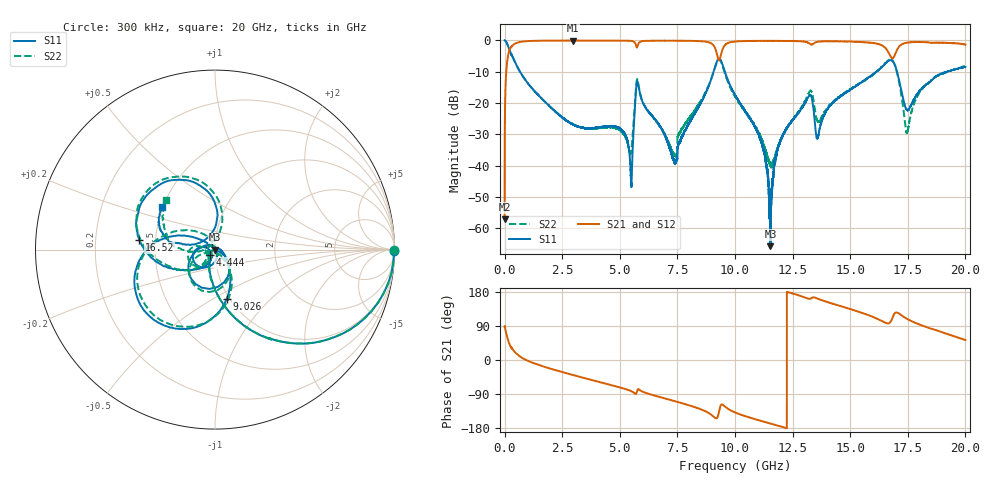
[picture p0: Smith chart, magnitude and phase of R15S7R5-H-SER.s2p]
!{R15S7R5}
!Johanson Technology Inc.
!www.johansontechnology.com
!Test Board Conditions:
!Substrate Type  RO4350B
!Substrate Thickness  20 mil
!Substrate Dk  3.66
!TL Type: GCPW
!TL Trace Width  34 mil
!TL Gap  10 mil
!Electrode orientation  Horizontal
!DUT TOPOLOGY	SERIES
!Mounting Pad LxW  26x52 mil
! Created Sat Feb  6 14:01:53 2021
# hz S ma R 50
! 2 Port Network Data from SP1.SP block
! freq  magS11  angS11  magS21  angS21  magS12  angS12  magS22  angS22
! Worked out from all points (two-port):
!   20001 points, 300 kHz to 20 GHz, reference 50 ohm
!   highest |S21| = -0.03 dB at 2.976 GHz (marker M1); lowest = -57.2 dB at 300 kHz (marker M2)
!   |S21| within 3 dB of the highest: 214.4 MHz to 9.166 GHz (8.952 GHz wide, 191 % of centre); 9.451 GHz to 16.6 GHz (7.147 GHz wide, 54.9 % of centre)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
!   lowest |S11| = -65.7 dB at 11.54 GHz (marker M3), VSWR 1.00, Z = 50 - j0.0291 ohm
!   |S11| at or under -10 dB: 669.7 MHz to 9.069 GHz (8.399 GHz wide, 172 % of centre); 9.562 GHz to 16.14 GHz (6.574 GHz wide, 51.2 % of centre); 17.03 GHz to 19.17 GHz (2.141 GHz wide, 11.8 % of centre)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
!   |S22| runs from -40.6 to 0.0 dB; largest |S21 - S12| = 0.015
!   S11 on the Smith chart (normalised r, x): 300 kHz: open; 4.444 GHz: 0.94, -0.06; 9.026 GHz: 0.97, -0.58; 16.52 GHz: 0.40, +0.05; 20 GHz: 0.50, +0.27
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300000  1 -0.3  0.001388 87.5  0.001436 92.7  0.9964 -0.2
1.093e8  0.8876 -28.8  0.4548 61.0  0.456 60.9  0.8886 -28.7
2.813e8  0.6005 -56.9  0.792 32.7  0.7922 32.6  0.6009 -56.7
2.9763e9  0.04502 -114.9  0.9963 -39.8  0.9951 -39.8  0.04561 -142.3
3.3343e9  0.04083 -116.1  0.9954 -45.6  0.9944 -45.7  0.04093 -152.6
4.4443e9  0.04278 -134.9  0.9921 -63.3  0.9923 -63.3  0.0412 -169.2
5.4763e9  0.007212 -144.1  0.9847 -81.7  0.9846 -81.7  0.01562 -98.2
5.7833e9  0.2123 -127.4  0.8351 -77.0  0.8359 -77.0  0.2248 -124.0
6.6673e9  0.04703 147.4  0.9893 -96.5  0.9894 -96.5  0.04743 -157.3
7.3993e9  0.01103 52.2  0.9881 -108.9  0.99 -108.9  0.01449 -96.4
9.0263e9  0.2807 -76.5  0.8676 -147.2  0.8695 -147.1  0.2803 -74.3
9.3913e9  0.4794 -159.3  0.5908 -118.5  0.5951 -118.6  0.4565 -161.7
1.00003e10  0.1348 149.9  0.9618 -138.4  0.9625 -138.4  0.1277 131.5
1.11013e10  0.02668 134.5  0.9842 -160.2  0.9832 -160.2  0.02902 111.7
1.15393e10  0.0005178 -145.8  0.9849 -167.8  0.9828 -167.7  0.01059 160.0
1.20213e10  0.02747 -65.4  0.9837 -176.1  0.9847 -176.0  0.02721 -126.5
1.33343e10  0.1204 -170.7  0.8591 163.6  0.8599 163.5  0.1494 -174.1
1.35923e10  0.02768 -137.9  0.9535 161.8  0.953 161.9  0.0513 -168.3
1.65213e10  0.4255 172.6  0.7647 98.6  0.7538 98.7  0.4322 169.3
1.66673e10  0.4712 156.1  0.6423 96.6  0.6285 97.0  0.4863 153.1
1.74703e10  0.07787 125.0  0.9241 108.3  0.9247 108.5  0.03387 138.1
2e10  0.3764 141.5  0.8566 52.7  0.8486 52.4  0.3908 134.1
